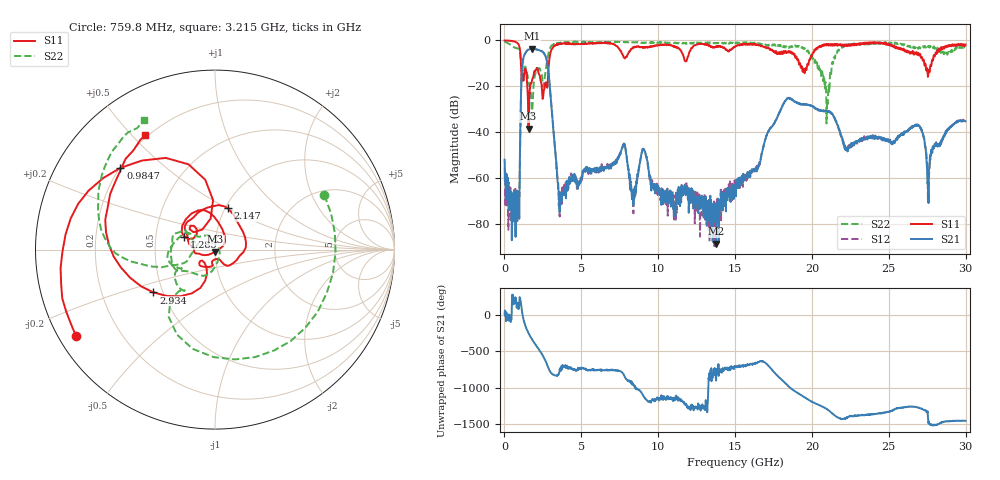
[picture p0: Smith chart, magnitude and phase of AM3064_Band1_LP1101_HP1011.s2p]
# Hz S DB R 50.0
!freq dBS11 angS11 dBS21 angS21 dBS12 angS12 dBS22 angS22
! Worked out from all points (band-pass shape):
!   1600 points, 10 MHz to 29.98 GHz, reference 50 ohm
!   highest |S21| = -3.58 dB at 1.791 GHz (marker M1); lowest = -88.4 dB at 13.77 GHz (marker M2)
!   |S21| within 3 dB of the highest: 1.283 GHz to 2.646 GHz (1.363 GHz wide, 69.4 % of centre)
!   lowest |S11| = -38.4 dB at 1.566 GHz (marker M3), VSWR 1.02, Z = 50.2 - j1.2 ohm
!   |S11| at or under -10 dB: 1.071 GHz to 2.894 GHz (1.822 GHz wide, 91.9 % of centre); 19.23 GHz to 19.79 GHz (558.7 MHz wide, 2.86 % of centre); 27.3 GHz to 27.78 GHz (478.8 MHz wide, 1.74 % of centre)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
!   |S22| runs from -36.1 to -0.4 dB; largest |S21 - S12| = 0.011
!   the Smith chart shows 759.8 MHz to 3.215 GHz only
!   S11 on the Smith chart (normalised r, x): 759.8 MHz: 0.05, -0.28; 984.7 MHz: 0.20, +0.36; 1.285 GHz: 0.70, +0.11; 2.147 GHz: 1.02, +0.51; 2.934 GHz: 0.44, -0.26; 3.215 GHz: 0.19, +0.55
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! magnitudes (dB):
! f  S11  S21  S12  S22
! 10 MHz  -0.1  -51.9  -55.6  -0.4
! 759.8 MHz  -0.8  -67.7  -67.1  -3.3
! 984.7 MHz  -3.1  -61.9  -60.1  -4.5
! 1.285 GHz  -14.6  -6.5  -6.5  -12.8
! 1.566 GHz  -38.4  -4.0  -3.9  -18.1
! 1.791 GHz  -17.4  -3.6  -3.6  -32.9
! 2.147 GHz  -12.3  -4.1  -4.1  -12.1
! 2.934 GHz  -7.6  -18.8  -18.8  -3.9
! 3.215 GHz  -2.5  -41.7  -41.5  -1.7
! 3.628 GHz  -1.4  -68.4  -71.7  -1.1
! 5.015 GHz  -1.4  -59.3  -59.1  -0.7
! 7.732 GHz  -6.8  -45.5  -45.5  -0.7
! 10 GHz  -2.1  -63.2  -66.6  -0.9
! 13.77 GHz  -2.8  -88.4  -87.7  -1.2
! 15 GHz  -2.7  -63.7  -66.4  -1.4
! 19.99 GHz  -6.8  -28.5  -28.5  -6.8
! 20.98 GHz  -1.7  -30.8  -30.7  -26.1
! 21.9 GHz  -2.1  -41.6  -41.8  -2.9
! 25 GHz  -1.5  -44.2  -43.3  -1.2
! 26.91 GHz  -5.4  -36.8  -36.7  -3.6
! 27.58 GHz  -13.4  -70.8  -63.7  -2.4
! 29.98 GHz  -1.8  -35.2  -34.9  -2.8
